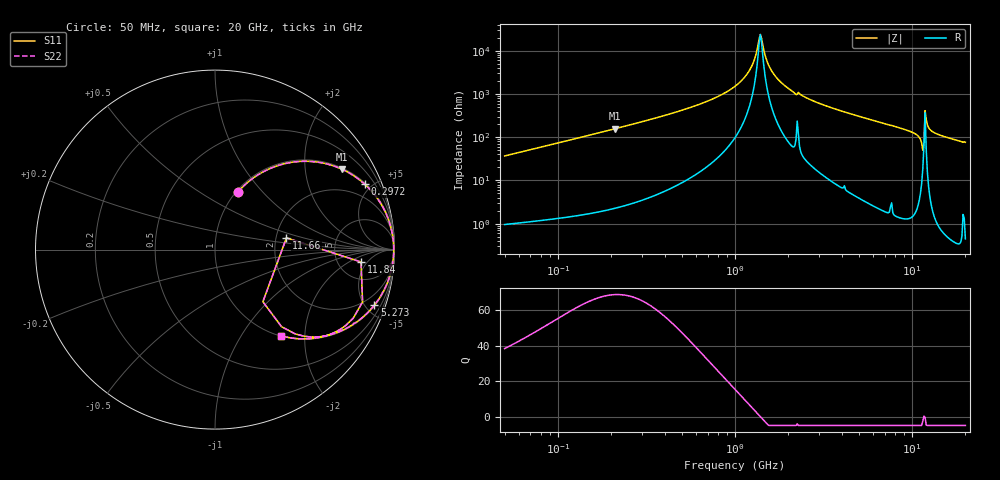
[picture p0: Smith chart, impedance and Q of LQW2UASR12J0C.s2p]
!Murata Part Number: LQW2UASR12J0C
!These Parameters are Measured in Series Mode Connection
!  o--[Z]--o
!Port1  Port2
!  o-------o
!Freq. Start=50[MHz] Stop=20[GHz], 401[Steps]
# Hz S RI R 50
!Freq.(Hz) S11(Real) S11(Imag) S21(Real) S21(Imag) S12(Real) S12(Imag) S22(Real) S22(Imag)
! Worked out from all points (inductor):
!   401 points, 50 MHz to 20 GHz, reference 50 ohm
!   read as one part in series: L = 117 nH near 51.52 MHz
!   highest Q = 68.9 at 210.6 MHz (marker M1), where L = 119 nH
!   self-resonance near 1.39 GHz
!   S11 on the Smith chart (normalised r, x): 50 MHz: 1.02, +0.74; 297.2 MHz: 1.07, +4.54; 5.273 GHz: 1.07, -5.72; 11.66 GHz: 2.28, +0.36; 11.84 GHz: 8.44, -3.48; 20 GHz: 1.01, -1.53
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5e7  0.1257 0.3187  0.8743 -0.3187  0.8743 -0.3187  0.1257 0.3187
1.364002e8  0.5029 0.4921  0.4971 -0.4921  0.4971 -0.4921  0.5029 0.4921
2.106029e8  0.7092 0.4469  0.2908 -0.4469  0.2908 -0.4469  0.7092 0.4469
2.972233e8  0.8337 0.3648  0.1663 -0.3648  0.1663 -0.3648  0.8337 0.3648
3.721004e8  0.891 0.3033  0.109 -0.3033  0.109 -0.3033  0.891 0.3033
6.87656e8  0.9735 0.1462  0.0265 -0.1462  0.0265 -0.1462  0.9735 0.1462
1e9  0.9914 0.0656  0.00865 -0.0656  0.00865 -0.0656  0.9914 0.0656
1.214974e9  0.9951 0.0267  0.00495 -0.0267  0.00495 -0.0267  0.9951 0.0267
1.390315e9  0.9958 0.000201  0.0042 -0.000201  0.0042 -0.000201  0.9958 0.000201
1.544007e9  0.9954 -0.0204  0.0046 0.0204  0.0046 0.0204  0.9954 -0.0204
1.714689e9  0.9941 -0.0413  0.00589 0.0413  0.00589 0.0413  0.9941 -0.0413
2.146657e9  0.9868 -0.0901  0.0132 0.0901  0.0132 0.0901  0.9868 -0.0901
2.728004e9  0.9764 -0.1377  0.0236 0.1377  0.0236 0.1377  0.9764 -0.1377
5.273168e9  0.8883 -0.309  0.1117 0.309  0.1117 0.309  0.8883 -0.309
7.442007e9  0.7837 -0.4069  0.2163 0.4069  0.2163 0.4069  0.7837 -0.4069
1.082228e10  0.5304 -0.4866  0.4696 0.4866  0.4696 0.4866  0.5304 -0.4866
1.131968e10  0.3705 -0.4293  0.6295 0.4293  0.6295 0.4293  0.3705 -0.4293
1.166392e10  0.3981 0.0653  0.6019 -0.0653  0.6019 -0.0653  0.3981 0.0653
1.183995e10  0.8134 -0.0687  0.1866 0.0687  0.1866 0.0687  0.8134 -0.0687
1.220001e10  0.7699 -0.3822  0.2301 0.3822  0.2301 0.3822  0.7699 -0.3822
1.295331e10  0.6494 -0.469  0.3506 0.469  0.3506 0.469  0.6494 -0.469
2e10  0.3684 -0.4795  0.6316 0.4795  0.6316 0.4795  0.3684 -0.4795
